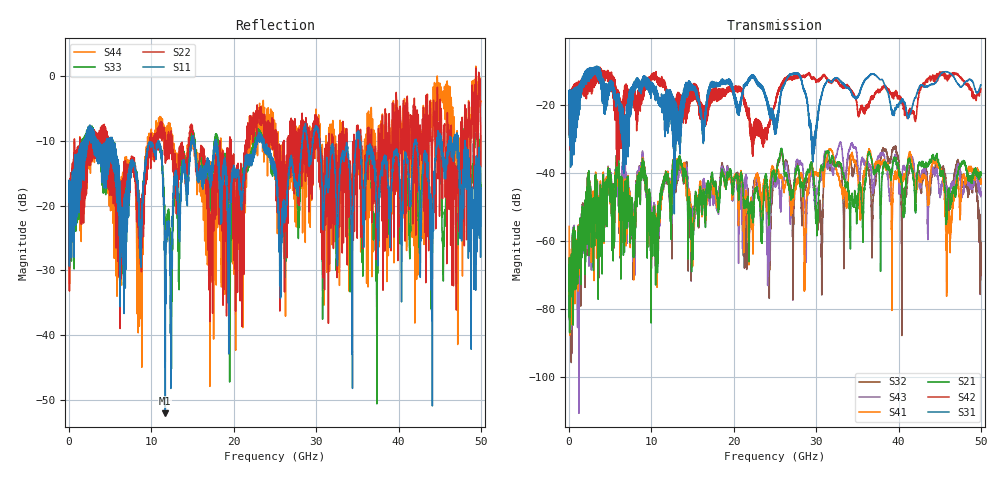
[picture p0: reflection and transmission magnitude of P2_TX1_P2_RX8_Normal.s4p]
!Keysight Technologies,N5225B,MY57041031,A.13.20.10
!Date: Friday, May 31, 2019 11:39:11
!Correction: S11(Full 4 Port(1,2,3,4))
!S12(Full 4 Port(1,2,3,4))
!S13(Full 4 Port(1,2,3,4))
!S14(Full 4 Port(1,2,3,4))
!S21(Full 4 Port(1,2,3,4))
!S22(Full 4 Port(1,2,3,4))
!S23(Full 4 Port(1,2,3,4))
!S24(Full 4 Port(1,2,3,4))
!S31(Full 4 Port(1,2,3,4))
!S32(Full 4 Port(1,2,3,4))
!S33(Full 4 Port(1,2,3,4))
!S34(Full 4 Port(1,2,3,4))
!S41(Full 4 Port(1,2,3,4))
!S42(Full 4 Port(1,2,3,4))
!S43(Full 4 Port(1,2,3,4))
!S44(Full 4 Port(1,2,3,4))
!S4P File: Measurements: <S11,S12,S13,S14>,
!<S21,S22,S23,S24>,
!<S31,S32,S33,S34>,
!<S41,S42,S43,S44>:
# Hz S  dB  R 50.0
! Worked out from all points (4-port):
!   5000 points, 10 MHz to 50 GHz, reference 50 ohm
!   strongest paths, dB at 10 MHz, 12.51 GHz, 25.01 GHz, 37.51 GHz, 50 GHz:
!     S31: -19.5, -17.3, -28.8, -12.1, -14.3
!     S42: -19.7, -21.3, -19.6, -16.0, -15.3
!     S21: -65.2, -41.2, -42.3, -37.9, -39.9
!     S41: -55.9, -40.3, -41.2, -37.3, -43.3
!     S43: -69.9, -43.6, -43.9, -35.1, -47.1
!     S32: -65.0, -45.6, -42.6, -37.6, -60.2
!   lowest |S11| = -52.1 dB at 11.69 GHz (marker M1), VSWR 1.00, Z = 49.8 - j0.166 ohm
!   |S11| at or under -10 dB: 5.36 GHz to 10.81 GHz (5.449 GHz wide, 67.4 % of centre); 17.89 GHz to 22.7 GHz (4.805 GHz wide, 23.7 % of centre); 35.31 GHz to 41.96 GHz (6.644 GHz wide, 17.2 % of centre)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
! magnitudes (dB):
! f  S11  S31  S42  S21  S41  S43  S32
! 10 MHz  -19.5  -19.5  -19.7  -65.2  -55.9  -69.9  -65.0
! 11.69 GHz  -52.1  -23.0  -13.7  -40.6  -40.4  -40.9  -41.1
! 24.19 GHz  -11.4  -20.1  -26.6  -48.6  -50.2  -58.4  -54.2
! 25.72 GHz  -34.0  -17.3  -14.0  -33.0  -41.0  -48.2  -34.1
! 30.52 GHz  -11.3  -18.6  -12.5  -39.4  -39.2  -41.8  -49.8
! 39.49 GHz  -11.6  -22.6  -17.4  -36.6  -42.0  -35.9  -33.0
! 50 GHz  -17.3  -14.3  -15.3  -39.9  -43.3  -47.1  -60.2
